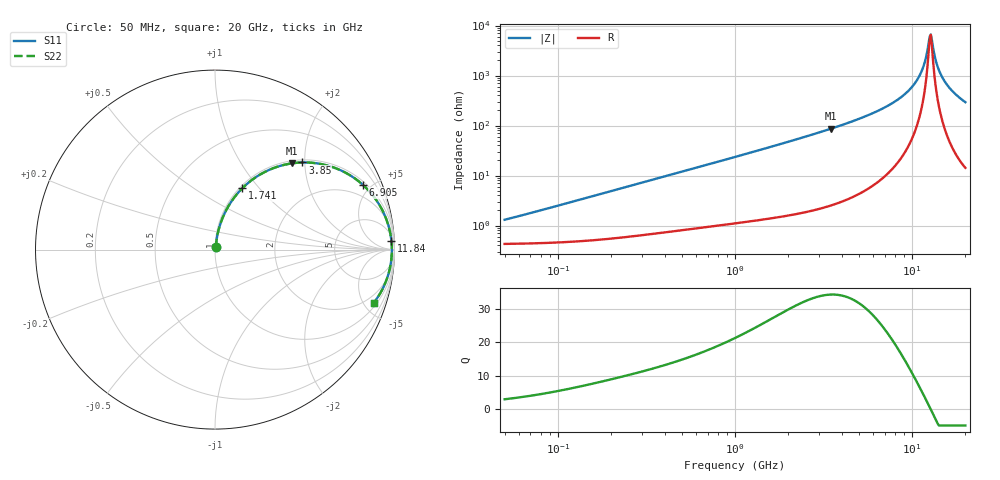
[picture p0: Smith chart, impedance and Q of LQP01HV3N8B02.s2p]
!Murata Part Number: LQP01HV3N8B02
!These Parameters are Measured in Series Mode Connection
!  o--[Z]--o
!Port1  Port2
!  o-------o
!Freq. Start=50[MHz] Stop=20[GHz], 401[Steps]
# Hz S RI R 50
!Freq.(Hz) S11(Real) S11(Imag) S21(Real) S21(Imag) S12(Real) S12(Imag) S22(Real) S22(Imag)
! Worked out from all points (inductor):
!   401 points, 50 MHz to 20 GHz, reference 50 ohm
!   read as one part in series: L = 3.91 nH near 53.09 MHz
!   highest Q = 34.3 at 3.467 GHz (marker M1), where L = 3.95 nH
!   self-resonance near 12.57 GHz
!   S11 on the Smith chart (normalised r, x): 50 MHz: 1.01, +0.02; 1.741 GHz: 1.03, +0.82; 3.85 GHz: 1.06, +1.95; 6.905 GHz: 1.18, +4.47; 11.84 GHz: 12, +37; 20 GHz: 1.28, -5.84
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5e7  0.00442 0.0122  0.9956 -0.0122  0.9956 -0.0122  0.00442 0.0122
1.364002e8  0.00595 0.033  0.994 -0.033  0.994 -0.033  0.00595 0.033
3.721004e8  0.0147 0.0871  0.9853 -0.0871  0.9853 -0.0871  0.0147 0.0871
1e9  0.0615 0.2179  0.9385 -0.2179  0.9385 -0.2179  0.0615 0.2179
1.740566e9  0.1528 0.3424  0.8472 -0.3424  0.8472 -0.3424  0.1528 0.3424
2.728004e9  0.3076 0.4467  0.6924 -0.4467  0.6924 -0.4467  0.3076 0.4467
3.466789e9  0.4275 0.4804  0.5725 -0.4804  0.5725 -0.4804  0.4275 0.4804
3.850025e9  0.4867 0.4854  0.5133 -0.4854  0.5133 -0.4854  0.4867 0.4854
5.194772e9  0.6661 0.4558  0.3339 -0.4558  0.3339 -0.4558  0.6661 0.4558
6.905011e9  0.8237 0.3611  0.1763 -0.3611  0.1763 -0.3611  0.8237 0.3611
7.442007e9  0.8589 0.3262  0.1411 -0.3262  0.1411 -0.3262  0.8589 0.3262
8.774992e9  0.9228 0.2375  0.0772 -0.2375  0.0772 -0.2375  0.9228 0.2375
1.004137e10  0.9595 0.1554  0.0405 -0.1554  0.0405 -0.1554  0.9595 0.1554
1.115139e10  0.9772 0.0875  0.0228 -0.0875  0.0228 -0.0875  0.9772 0.0875
1.183995e10  0.9829 0.0476  0.0171 -0.0476  0.0171 -0.0476  0.9829 0.0476
1.238412e10  0.985 0.0174  0.015 -0.0174  0.015 -0.0174  0.985 0.0174
1.276073e10  0.9854 -0.00282  0.0146 0.00282  0.0146 0.00282  0.9854 -0.00282
1.295331e10  0.9853 -0.013  0.0147 0.013  0.0147 0.013  0.9853 -0.013
1.396067e10  0.9814 -0.0637  0.0186 0.0637  0.0186 0.0637  0.9814 -0.0637
1.504638e10  0.9721 -0.1142  0.0279 0.1142  0.0279 0.1142  0.9721 -0.1142
1.696185e10  0.9456 -0.1935  0.0544 0.1935  0.0544 0.1935  0.9456 -0.1935
2e10  0.8839 -0.2969  0.1161 0.2969  0.1161 0.2969  0.8839 -0.2969
